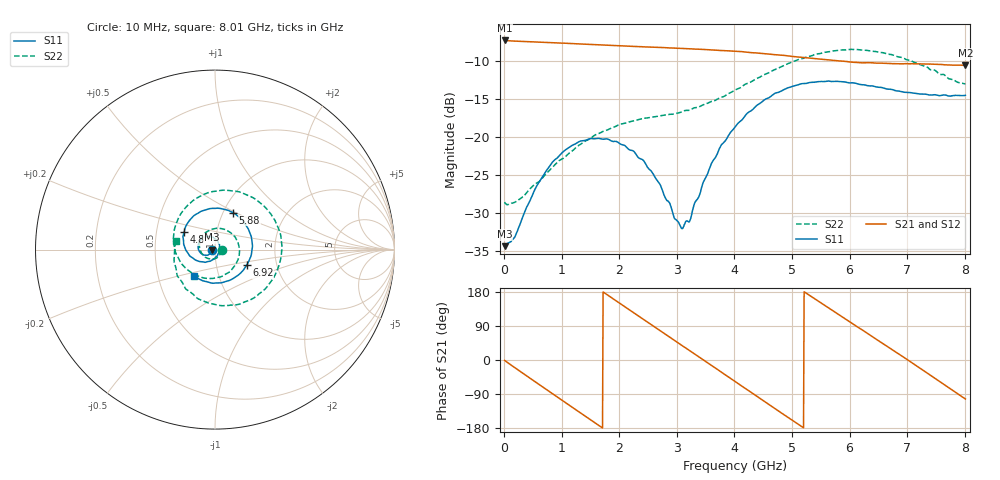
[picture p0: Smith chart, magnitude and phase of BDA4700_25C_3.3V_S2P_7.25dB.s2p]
!Agilent Technologies,E5071B,MY42404982,A.09.10
!Date: Mon Oct 20 18:06:02 2025
!Data & Calibration Information:
!Freq	S11:SOLT2(ON)	S21:SOLT2(ON)	S12:SOLT2(ON)	S22:SOLT2(ON)
# Hz S RI R 50
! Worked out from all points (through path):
!   801 points, 10 MHz to 8.01 GHz, reference 50 ohm
!   highest |S21| = -7.36 dB at 10 MHz (marker M1); lowest = -10.6 dB at 8.01 GHz (marker M2)
!   group delay of S21, straight-line fit = 285 ps
!   lowest |S11| = -34.4 dB at 10 MHz (marker M3), VSWR 1.04, Z = 48.1 - j0.0907 ohm
!   |S11| at or under -10 dB: start of sweep to end of sweep
!   |S22| runs from -29.0 to -8.5 dB; largest |S21 - S12| = 0.005
!   S11 on the Smith chart (normalised r, x): 10 MHz: 0.96, -0.00; 4.8 GHz: 0.69, +0.14; 5.88 GHz: 1.11, +0.48; 6.92 GHz: 1.40, -0.26; 8.01 GHz: 0.76, -0.23
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1e7  -0.019 -0.000941  0.4283 -0.00927  0.4282 -0.00959  0.037 -0.00276
3.3e8  -0.0237 -0.0183  0.3445 -0.2437  0.3443 -0.2438  0.0242 -0.0321
7.1e8  -0.0481 -0.0318  0.1063 -0.4024  0.1062 -0.4025  -0.0185 -0.0527
1.02e9  -0.0757 -0.0229  -0.1242 -0.3921  -0.1244 -0.3921  -0.0626 -0.035
1.35e9  -0.0936 0.00584  -0.3198 -0.2499  -0.3199 -0.25  -0.087 0.0226
1.64e9  -0.0893 0.0387  -0.3975 -0.0552  -0.3977 -0.0551  -0.0664 0.0807
1.93e9  -0.0669 0.0646  -0.3674 0.1496  -0.3672 0.1497  -0.00541 0.1161
2.32e9  -0.0224 0.0701  -0.1812 0.3458  -0.181 0.3461  0.0907 0.0916
2.68e9  0.0144 0.0481  0.0634 0.3804  0.0628 0.3803  0.1363 0.000445
3.1e9  0.0243 -0.00508  0.3026 0.2291  0.3007 0.2309  0.09 -0.1153
3.23e9  0.0185 -0.0212  0.3448 0.1536  0.345 0.153  0.0564 -0.1385
3.54e9  -0.0127 -0.0563  0.3691 -0.0514  0.369 -0.0522  -0.0431 -0.1603
4.01e9  -0.0969 -0.0627  0.2006 -0.3034  0.2009 -0.3032  -0.1857 -0.0788
4.39e9  -0.1603 -0.00692  -0.0357 -0.3523  -0.0359 -0.3532  -0.2318 0.0659
4.8e9  -0.1723 0.0976  -0.2558 -0.229  -0.254 -0.2302  -0.1626 0.2355
5.35e9  -0.0675 0.217  -0.3168 0.0805  -0.317 0.0788  0.0957 0.3268
5.88e9  0.1002 0.2058  -0.1199 0.2894  -0.1199 0.2887  0.334 0.1625
6.27e9  0.186 0.1143  0.0818 0.2941  0.0861 0.292  0.3644 -0.0604
6.68e9  0.204 -0.0175  0.2532 0.1648  0.254 0.1642  0.2393 -0.2524
6.92e9  0.1763 -0.0875  0.2972 0.0479  0.2968 0.0463  0.1187 -0.3079
7.48e9  0.0359 -0.1849  0.1993 -0.2221  0.1993 -0.2229  -0.1638 -0.2181
8.01e9  -0.1164 -0.1461  -0.0656 -0.2862  -0.0649 -0.2866  -0.2166 0.0467
